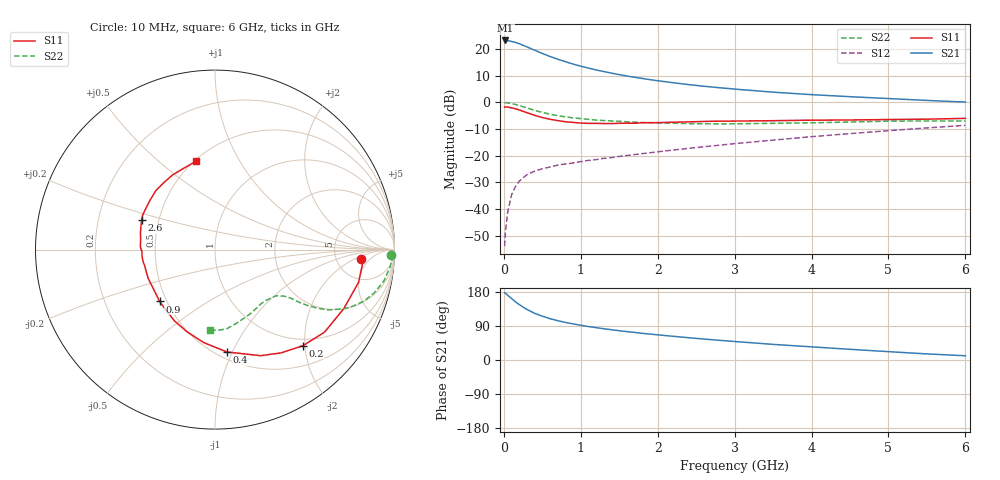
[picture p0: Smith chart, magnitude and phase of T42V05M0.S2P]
! Infineon Technologies  Discrete & RF Semiconductors
! BFR182T
! Si NPN RF Bipolar Junction Transistor in SC75
! VCE = 2 V  IC = 5 mA
! Common Emitter S-Parameters:  October  1999
# GHz  S  MA  R  50
!  f  S11  S21  S12  S22
! GHz  MAG  ANG  MAG  ANG  MAG  ANG  MAG  ANG
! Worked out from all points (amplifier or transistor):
!   36 points, 10 MHz to 6 GHz, reference 50 ohm
!   highest |S21| = 23.3 dB at 20 MHz (marker M1)
!   |S21| within 3 dB of that: start of sweep to 347.1 MHz
!   unconditionally stable (mu >= 1): 1.354 GHz to 4.01 GHz
!   at 250 MHz: K = 0.29, MSG = 24.9 dB, |S12| = -28.3 dB
!   at 1.4 GHz: K = 1.02, MAG = 15.0 dB, |S12| = -20.7 dB
!   at 6 GHz: K = 0.84, MSG = 4.4 dB, |S12| = -8.6 dB
!   lowest NFmin = 1.20 dB at 450 MHz
!   S11 on the Smith chart (normalised r, x): 10 MHz: 9.01, -2.76; 200 MHz: 0.87, -1.96; 400 MHz: 0.56, -0.95; 900 MHz: 0.46, -0.32; 2.6 GHz: 0.40, +0.16; 6 GHz: 0.51, +0.67
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0.01  0.816 -3.6  14.57 177.4  0.002 83.7  0.983 -1.9
0.02  0.8287 -3.8  14.63 176.6  0.0036 91.8  0.9894 -2.2
0.05  0.8206 -12.8  14.52 170.8  0.0087 87.5  0.9812 -5.5
0.1  0.7895 -24.6  14.03 162.3  0.0183 77.8  0.9569 -10.6
0.15  0.7642 -37.0  13.46 153.7  0.0261 72.7  0.9192 -15.2
0.2  0.726 -47.5  12.72 146.3  0.0332 68.1  0.8788 -19.0
0.25  0.6835 -57.3  11.88 139.6  0.0386 63.0  0.8319 -22.2
0.3  0.6436 -66.7  11.08 133.5  0.0439 60.9  0.7903 -24.7
0.4  0.5743 -83.3  9.604 123.3  0.0514 56.2  0.7111 -28.2
0.5  0.5222 -96.8  8.349 115.6  0.057 53.2  0.6508 -29.9
0.6  0.4838 -108.8  7.316 109.1  0.0613 51.6  0.6032 -31.1
0.7  0.457 -119.5  6.509 103.8  0.0667 51.7  0.5656 -31.8
0.8  0.4351 -128.6  5.84 99.1  0.0699 51.3  0.5366 -32.3
0.9  0.4227 -136.9  5.269 95.3  0.0731 51.5  0.5136 -32.5
1.1  0.4052 -151.1  4.427 88.2  0.0817 53.1  0.4817 -33.4
1.6  0.4082 -175.3  3.144 74.9  0.1009 56.2  0.434 -36.3
2.2  0.4261 167.2  2.35 62.5  0.1279 59.5  0.4079 -42.4
2.6  0.4402 158.3  2.02 55.3  0.1475 60.8  0.3982 -47.4
3.5  0.455 142.5  1.562 41.2  0.1963 61.1  0.4062 -59.6
4.5  0.4692 127.9  1.285 28.2  0.2603 58.5  0.4292 -74.5
5.5  0.4864 110.4  1.094 16.1  0.3333 53.7  0.45 -87.9
6  0.5033 102.1  1.018 11.2  0.3724 50.3  0.4483 -93.6
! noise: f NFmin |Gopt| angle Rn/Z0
0.45  1.2  0.27  37  0.3
0.9  1.3  0.25  75  0.23
1.8  1.9  0.21  145  0.2
